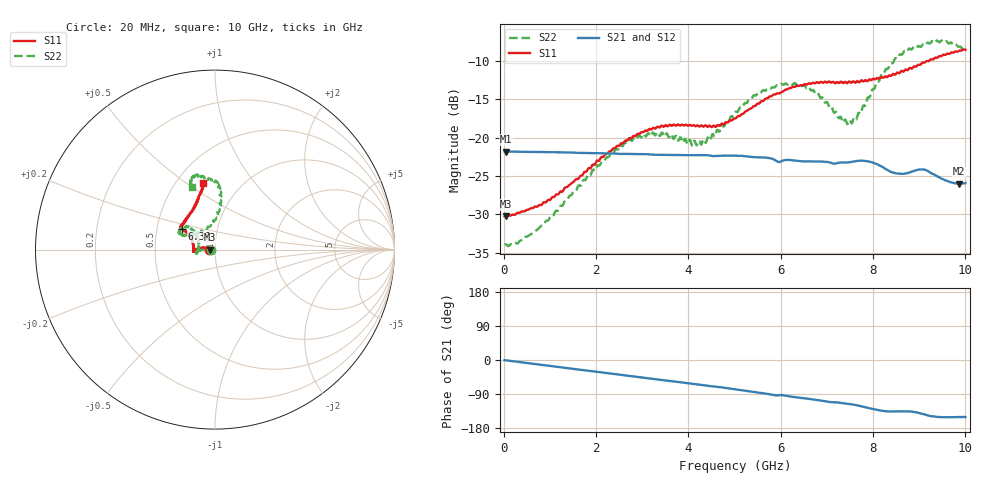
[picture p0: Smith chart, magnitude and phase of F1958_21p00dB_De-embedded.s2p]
! Integrated Device Technology
! Corporate Headquarters
! 6024 Silver Creek Valley Road
! San Jose, CA 95138  USA
! Phone:  1-408-284-8200
! Toll Free:  1-800-223-1366
! Webpage:  http://www.idt.com/
! Timing and RF Division
! 515 Groton Road, Suite 102
! Westford, MA 01886-6024
! Device:  F1958
! Description: 7-bit 0.25 dB Digital Step Attenuator
! Frequency:  0.001 -  6.000 GHz
! Package:  4x4 mm Thin QFN Plastic Package: 24 pin
! Ports:  2 RF, 12 DC
!  Pin  1  = D0
!  Pin  2  = VDD
!  Pin  3  = VMODE
!  Pin  4  = GND
!  Pin  5  = RF1  =  Port 1
!  Pin  6  = GND
!  Pin  7  = GND
!  Pin  8  = GND
!  Pin  9  = GND
!  Pin 10  = GND
!  Pin 11  = GND
!  Pin 12  = GND
!  Pin 13  = GND
!  Pin 14  = RF2  =  Port 2
!  Pin 15  = GND
!  Pin 16  = LE
!  Pin 17  = CLK
!  Pin 18  = DATA
!  Pin 19  = D6
!  Pin 20  = D5
!  Pin 21  = D4
!  Pin 22  = D3
!  Pin 23  = D2
!  Pin 24  = D1
! State:  84
! Atten State:  21.00 dB
! Voltage:  +3.30 Volts
! Current:  0.258 mA
! Data:  The device was measured on a F1958 evaluation board which has
!  individual transmission lines to the RF pins.  Data was collected
!  using a calibrated network analyzer.  The evaluation board was
!  de-embedded using Automatic Fixture Removal (AFR).
!  The reference plane is the edge of the package pin.
! Misc:
!  Action Tracker AT0419
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# GHz S dB R 50
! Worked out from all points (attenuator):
!   500 points, 20 MHz to 10 GHz, reference 50 ohm
!   highest |S21| = -21.81 dB at 40 MHz (marker M1); lowest = -26.0 dB at 9.86 GHz (marker M2)
!   lowest |S11| = -30.3 dB at 40 MHz (marker M3), VSWR 1.06, Z = 47 - j0.0418 ohm
!   |S11| at or under -10 dB: start of sweep to 9.206 GHz
!   |S22| runs from -34.2 to -7.3 dB; largest |S21 - S12| = 0.00038
!   S11 on the Smith chart (normalised r, x): 20 MHz: 0.94, -0.00; 6.36 GHz: 0.67, +0.16; 10 GHz: 0.68, +0.58
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0.02  -30.26 -178.9  -21.81 -0.4  -21.81 -0.4  -33.96 -177.9
0.04  -30.29 -179.2  -21.81 -0.7  -21.81 -0.7  -33.90 -177.1
0.32  -29.81 175.1  -21.84 -5.1  -21.84 -5.1  -33.71 178.4
0.72  -29.03 172.6  -21.87 -11.3  -21.87 -11.3  -32.03 179.4
1.7  -24.93 170.9  -22.00 -26.2  -21.99 -26.2  -25.85 178.8
2.6  -20.64 176.9  -22.12 -40.0  -22.11 -40.0  -20.86 -176.4
3.36  -18.66 -175.5  -22.25 -51.8  -22.24 -51.9  -19.61 -168.2
4.24  -18.57 -178.8  -22.29 -65.1  -22.30 -65.1  -20.45 169.8
4.52  -18.57 174.2  -22.41 -69.6  -22.43 -69.7  -19.52 154.3
5.02  -17.51 160.9  -22.35 -77.3  -22.36 -77.3  -16.63 139.6
5.58  -15.25 150.7  -22.58 -86.8  -22.60 -86.8  -14.06 140.0
6.36  -13.23 148.2  -23.03 -98.9  -23.05 -98.9  -13.18 153.6
6.68  -12.89 146.7  -23.10 -103.6  -23.11 -103.5  -13.83 155.0
7.32  -12.72 141.5  -23.26 -113.6  -23.27 -113.5  -17.58 134.8
7.5  -12.72 138.4  -23.21 -116.3  -23.21 -116.3  -17.74 116.7
7.68  -12.69 135.5  -23.03 -120.2  -23.02 -120.2  -16.81 99.0
8.34  -11.90 119.3  -24.32 -135.7  -24.31 -135.8  -10.85 83.1
8.68  -11.27 112.6  -24.71 -135.3  -24.71 -135.3  -8.69 87.6
9.04  -10.40 107.2  -24.17 -141.3  -24.17 -141.3  -8.14 95.4
9.26  -9.76 105.0  -24.65 -148.1  -24.63 -148.2  -7.52 100.5
9.86  -8.67 100.1  -26.02 -150.4  -26.06 -150.4  -8.15 109.6
10  -8.54 100.1  -25.93 -150.6  -25.99 -150.4  -8.64 110.5
